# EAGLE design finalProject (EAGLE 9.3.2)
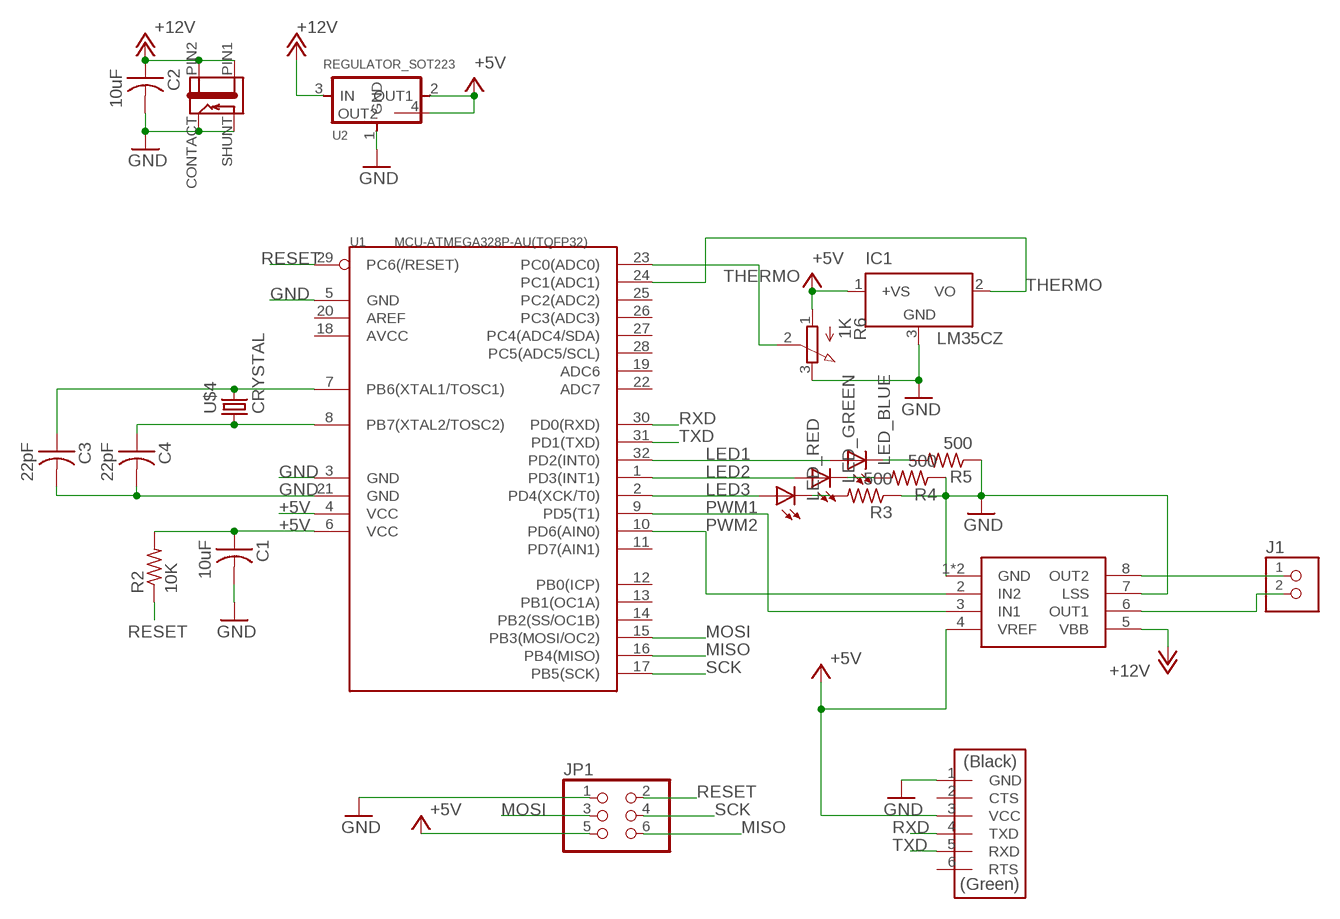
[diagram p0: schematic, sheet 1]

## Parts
C1  10uF  CAP-US1206FAB  [C1206FAB]
C2  10uF  CAP-US1206FAB  [C1206FAB]
C3  22pF  CAP-US1206FAB  [C1206FAB]
C4  22pF  CAP-US1206FAB  [C1206FAB]
IC1  LM35CZ  [TO92]
J1  TERM-1X02-FABLAB  [ED555DS-2DS]
J2  JACK-2.1MM  [PJ-002AH-SMT]
JP1  PINHD-2X3-SMD  [2X03SMD]
LED_BLUE  LEDFAB1206  [LED1206FAB]
LED_GREEN  LEDFAB1206  [LED1206FAB]
LED_RED  LEDFAB1206  [LED1206FAB]
R2  10K  RES-US1206FAB  [R1206FAB]
R3  500  RES-US1206FAB  [R1206FAB]
R4  500  RES-US1206FAB  [R1206FAB]
R5  500  RES-US1206FAB  [R1206FAB]
R6  1K  3RP/1610N  [3RP/1610N]
U1  MCU-ATMEGA328P-AU(TQFP32)  [TQFP32-0.8-7X7MM]
U2  REGULATOR_SOT223  [SOT223]
U$1  A4953-H-BRIDGE-MOTOR-DRIVER-PAD  [SOIC8_PAD]
U$2  FTDI-SMD-HEADER  [1X06SMD]
U$4  CRYSTAL  [2-SMD-5X3MM]

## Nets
+5V: C1.1 IC1.1(+VS) JP1.5 R2.2 R6.1(A) U1.4(VCC) U1.6(VCC) U2.2(OUT1) U2.4(OUT2) U$1.4(VREF) U$2.3(VCC)
+12V: C2.1 J2.PIN1 J2.PIN2 U2.3(IN) U$1.5(VBB)
GND: C1.2 C2.2 C3.2 C4.2 IC1.3(GND) J2.CONTACT J2.SHUNT JP1.1 R3.1 R4.1 R5.1 R6.3(E) U1.3(GND) U1.5(GND) U1.21(GND) U2.1(GND) U$1.1(GND) U$1.7(LSS) U$1.GND U$2.1(GND)
LED1: LED_BLUE.1(A) U1.32(PD2(INT0))
LED2: LED_GREEN.1(A) U1.1(PD3(INT1))
LED3: LED_RED.1(A) U1.2(PD4(XCK/T0))
MISO: JP1.6 U1.16(PB4(MISO))
MOSI: JP1.3 U1.15(PB3(MOSI/OC2))
N$1: R6.2(S) U1.23(PC0(ADC0))
N$2: LED_RED.2(C) R3.2
N$3: LED_BLUE.2(C) R5.2
N$4: C3.1 U1.7(PB6(XTAL1/TOSC1)) U$4.P$2
N$5: C4.1 U1.8(PB7(XTAL2/TOSC2)) U$4.P$1
N$6: LED_GREEN.2(C) R4.2
N$7: J1.1 U$1.8(OUT2)
N$8: J1.2 U$1.6(OUT1)
PWM1: U1.9(PD5(T1)) U$1.3(IN1)
PWM2: U1.10(PD6(AIN0)) U$1.2(IN2)
RESET: JP1.2 R2.1 U1.29(PC6(/RESET))
RXD: U1.30(PD0(RXD)) U$2.4(TXD)
SCK: JP1.4 U1.17(PB5(SCK))
THERMO: IC1.2(VO) U1.24(PC1(ADC1))
TXD: U1.31(PD1(TXD)) U$2.5(RXD)
Unconnected: U1.11(PD7(AIN1)) U1.12(PB0(ICP)) U1.13(PB1(OC1A)) U1.14(PB2(SS/OC1B)) U1.18(AVCC) U1.19(ADC6) U1.20(AREF) U1.22(ADC7) U1.25(PC2(ADC2)) U1.26(PC3(ADC3)) U1.27(PC4(ADC4/SDA)) U1.28(PC5(ADC5/SCL)) U$2.2(CTS) U$2.6(RTS)

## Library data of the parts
C1-C4 = fab:CAP-US
IC1 = lm35:LM35: Single-Supply Centigrade Temperature Sensor Vout = (10mV/°C x Temp °C) +5mmmV Source: http://www.national.com/ds/LM/LM35.pdf
J1 = fab:TERM-1X02: 3.5mm terminal block, 2 positions ED555-2DS as found in the fablab inventory.
J2 = fab:JACK-2.1MM: SMD DC power jack PJ-002AH-SMT As found in the fablab inventory. Made by Zaerc.
JP1 = fab:PINHD-2X3-SMD: PIN HEADER
LED_BLUE LED_GREEN LED_RED = fab:LED: LED
R2-R5 = fab:RES-US: Resistor (US Symbol)
R6 = pot:3RP/1610N: 16mm Potentiometer one level Source: http://www.alphapotentiometers.net/html/16mm_pot_2.html
U1 = MCU-ATMEGA328P-AU_TQFP32_:MCU-ATMEGA328P-AU(TQFP32): 310010049; AVAILABILITY: Unavailable; DESCRIPTION: Microcontroller Mcu, 8 Bit, Atmega, 20mhz, Tqfp-32; MF: Microchip; MP: ATMEGA328P-AU; PACKAGE: TQFP-32 Microchip; PRICE: None
U2 = fab:REGULATOR_SOT223
U$1 = fab:A4953-H-BRIDGE-MOTOR-DRIVER-PAD
U$2 = fab:FTDI-SMD-HEADER
U$4 = fab:CRYSTAL

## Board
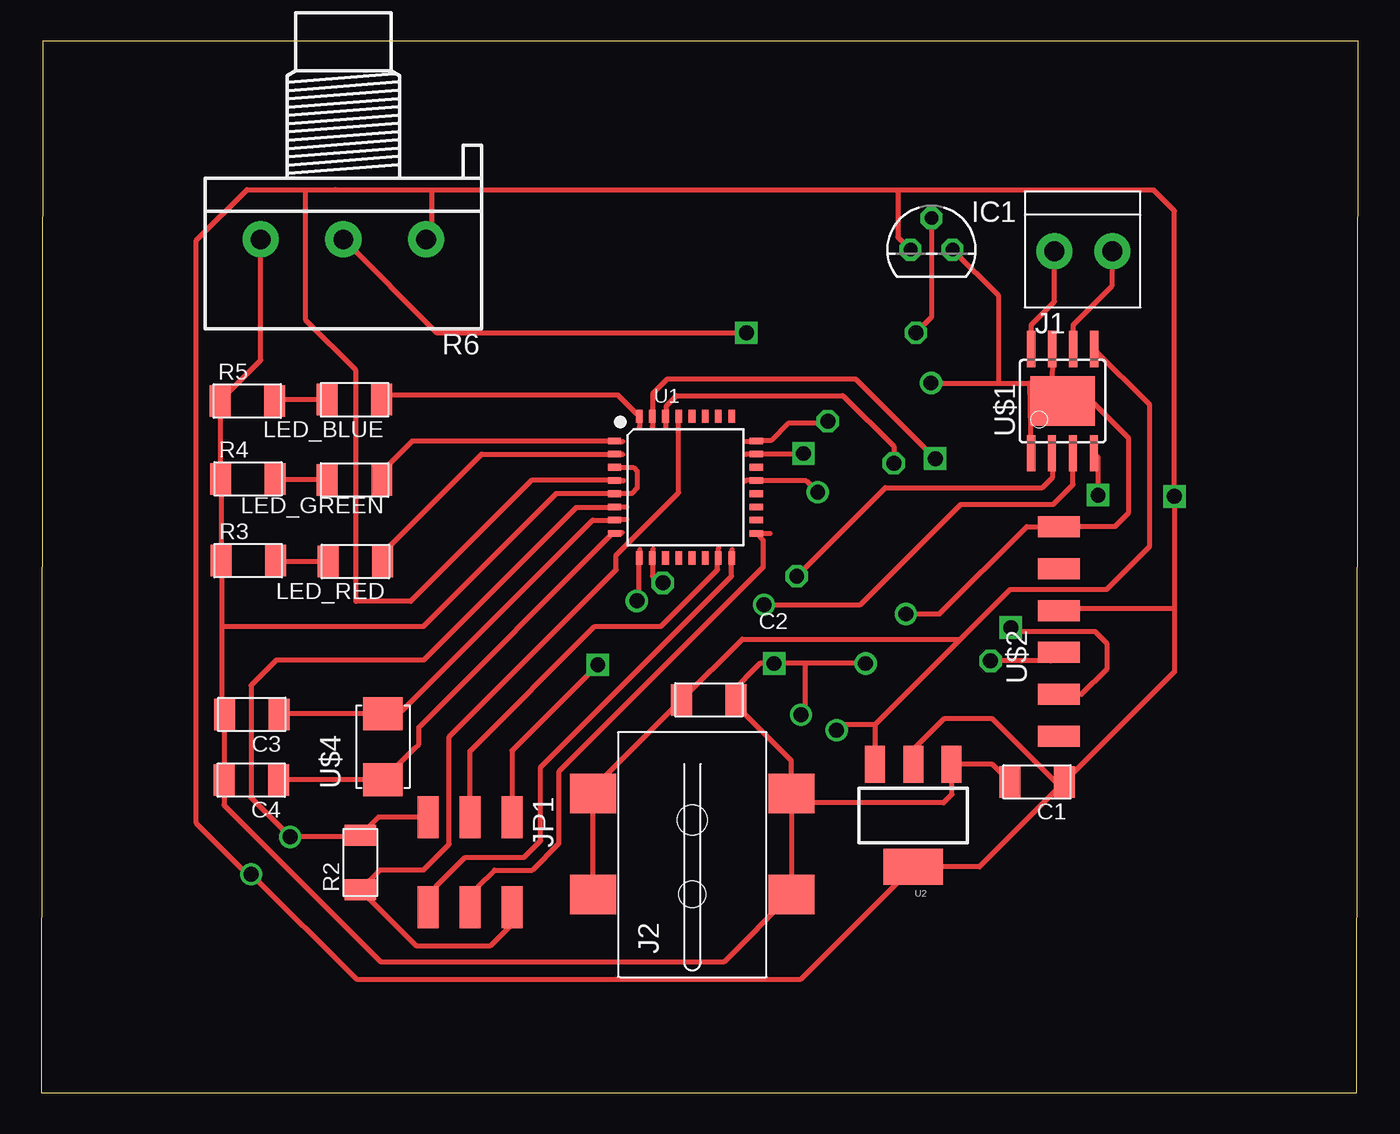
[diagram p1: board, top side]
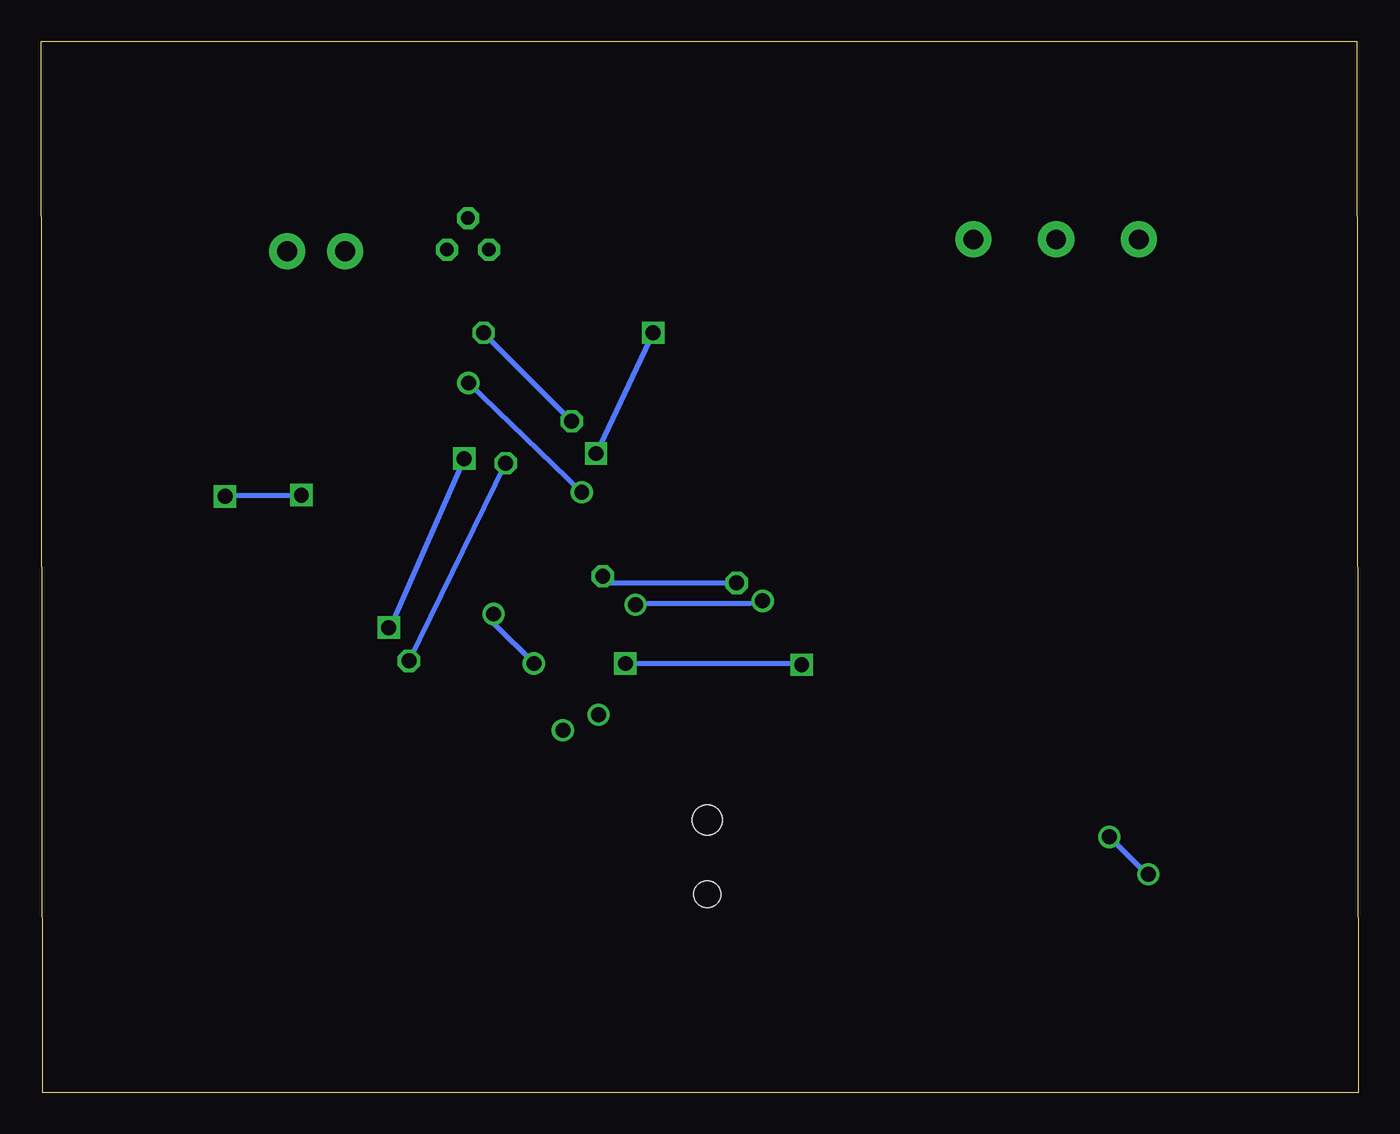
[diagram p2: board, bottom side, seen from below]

Size 79.7 x 63.6 mm. Coordinates in mm from the lower left corner, seen from the top.
Outline: 0,0 79.6,0 79.7,63.6 0.1,63.6 0,0
Copper layers (1*16): Top 0.035mm / dielectric 1.5mm / Bottom 0.035mm
Design rules "default *": minimum track width 6mil, minimum drill 0.35mm, track to track 0.4mm, track to pad 0.4mm, pad to pad 0.4mm, via to via 0.4mm, smd to smd 0.4mm, copper to edge 40mil, drill to drill 6mil, minimum pad ring 10mil, minimum via ring 8mil, stop-mask expansion 4mil, vias tented up to drill 0mil, thermal gap 10mil

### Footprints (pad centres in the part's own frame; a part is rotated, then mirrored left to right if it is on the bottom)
C1206FAB = smd 1.27 x 1.905: 1 -1.651,0; 2 1.651,0
TO92 = drill 0.813 octagon: 1 -1.27,0; 2 0,1.905; 3 1.27,0
ED555DS-2DS = drill 1.2 pad 2.184: 1 1.8,0; 2 -1.7,0
PJ-002AH-SMT = smd 2.4 x 2.8: CONTACT -2.4,-6; PIN1 3.7,6; PIN2 -2.4,6; SHUNT 3.7,-6 | hole 1.6: -2.4,0 | hole 1.8: 2.1,0
2X03SMD = smd 2.54 x 1.27: 1 -2.54,2.54; 2 2.92,2.54; 3 -2.54,0; 4 2.92,0; 5 -2.54,-2.54; 6 2.92,-2.54
LED1206FAB = smd 1.27 x 1.905: 1 -1.651,0; 2 1.651,0
R1206FAB = smd 1.27 x 1.905: 1 -1.651,0; 2 1.651,0
3RP/1610N = drill 1.2 pad 2.184: 1 -5,0; 2 0,0; 3 5,0
TQFP32-0.8-7X7MM = smd 0.8 x 0.4: 1 -4.293,2.8; 2 -4.293,2; 3 -4.293,1.2; 4 -4.293,0.4; 5 -4.293,-0.4; 6 -4.293,-1.2; 7 -4.293,-2; 8 -4.293,-2.8; 17 4.293,-2.8; 18 4.293,-2; 19 4.293,-1.2; 20 4.293,-0.4; 21 4.293,0.4; 22 4.293,1.2; 23 4.293,2; 24 4.293,2.8 | smd 0.4 x 0.8: 9 -2.8,-4.293; 10 -2,-4.293; 11 -1.2,-4.293; 12 -0.4,-4.293; 13 0.4,-4.293; 14 1.2,-4.293; 15 2,-4.293; 16 2.8,-4.293; 25 2.8,4.293; 26 2,4.293; 27 1.2,4.293; 28 0.4,4.293; 29 -0.4,4.293; 30 -1.2,4.293; 31 -2,4.293; 32 -2.8,4.293
SOT223 = smd 1.219 x 2.235: 1 -2.311,-3.099; 2 0,-3.099; 3 2.311,-3.099 | smd 3.6 x 2.2: 4 0,3.099
SOIC8_PAD = smd 0.5 x 2.2: 1 -1.905,-3.154; 2 -0.645,-3.154; 3 0.625,-3.154; 4 1.895,-3.154; 5 1.905,3.154; 6 0.635,3.154; 7 -0.635,3.154; 8 -1.905,3.154 | smd 3.886 x 2.997: GND 0,0
1X06SMD = smd 2.54 x 1.27: 1 0,6.35; 2 0,3.81; 3 0,1.27; 4 0,-1.27; 5 0,-3.81; 6 0,-6.35
2-SMD-5X3MM = smd 2 x 2.4: P$1 -2,0; P$2 2,0

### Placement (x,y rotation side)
C1  60.26,18.79 180 top
C2  40.4,23.76 0 top
C3  12.74,22.88 180 top
C4  12.71,18.9 180 top
IC1  53.87,50.99 0 top
J1  63.12,50.9 180 top
J2  39.4,14.39 90 top
JP1  25.94,14.12 270 top
LED_BLUE  18.96,41.92 180 top
LED_GREEN  18.96,37.06 180 top
LED_RED  19.01,32.13 180 top
R2  19.31,13.91 90 top
R3  12.52,32.19 0 top
R4  12.51,37.13 0 top
R5  12.47,41.84 0 top
R6  18.28,51.61 180 top
U1  38.98,36.63 0 top
U2  52.77,16.76 180 top
U$1  61.81,41.83 0 top
U$2  61.58,27.89 0 top
U$4  20.68,20.92 90 top

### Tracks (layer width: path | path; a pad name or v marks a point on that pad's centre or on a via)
+5V  (via drill 0.9)
  Top 0.305: IC1.1 51.84,51.76 51.84,54.61 23.62,54.61 | U2.2 52.6,20.02 52.6,20.57 54.64,22.61 57.57,22.61 61.38,18.79 C1.1 | JP1.5 20.4,16.66 R2.2 | C1.1 56.78,13.66 U2.4 45.97,6.86 19.07,6.86 v12.71,13.22 | 17.78,54.61 17.8,54.63 12.45,54.63 9.38,51.56 9.38,16.3 12.46,13.22 v12.71,13.22 | 17.78,54.61 16,54.61 16,46.74 19.05,43.69 19.05,29.72 22.35,29.72 29.66,37.03 U1.4 35.21,37.03 35.23,37.01 | 17.78,54.61 23.62,54.61 | 23.62,54.61 23.62,51.95 R6.1 | 51.59,54.61 67.31,54.61 68.58,53.34 v68.58,36.07 68.58,29.29 | C1.1 68.58,25.46 68.58,29.29 | U$2.3 61.71,29.29 68.58,29.29 | U$1.4 63.96,38.43 v63.96,36.14 | 19.11,15.37 R2.2 | 19.24,15.49 R2.2 | v12.7,13.21 v12.71,13.22 | R2.2 19.21,15.47 v15.06,15.47 12.7,17.83 12.7,24.64 14.22,26.16 23.14,26.16 32.36,35.38 34.64,35.38 U1.6 35.43,35.43
  Bottom 0.305: v68.58,36.07 68.5,36.14 v63.96,36.14 | v15.06,15.47 12.8,13.21 v12.7,13.21
+12V  (via drill 0.9)
  Top 0.305: J2.PIN2 J2.PIN1 33.4,18.41 C2.1 42.42,27.43 55.63,27.43 | U$1.5 67.06,41.65 67.06,33.02 64.47,30.43 58.62,30.43 55.63,27.43 | 50.46,22.27 U2.3 | 55.63,27.43 50.46,22.27 | 50.46,22.27 48.48,22.27 v48.13,21.92
GND  (via drill 0.9)
  Top 0.305: 11.06,22.85 C3.2 11.19,22.78 | 11.06,22.85 C4.2 11.06,17.39 20.52,7.92 41.34,7.92 J2.CONTACT | R6.3 13.28,44.3 R5.1 10.86,41.8 R4.1 10.87,37.12 R3.1 10.92,32.13 10.92,28.19 | IC1.3 57.91,48.23 57.91,42.93 | J2.SHUNT 45.4,20.08 41.88,23.6 C2.2 | C2.2 41.67,24.14 43.48,25.96 v44.35,25.96 44.37,25.98 46.23,25.98 | C2.2 | J2.CONTACT 44.54,12.85 | U2.1 55.48,19.86 | U2.1 55.12,19.82 55.12,18.03 54.61,17.53 45.96,17.53 J2.SHUNT | U$2.1 61.38,34.04 | 11.06,22.85 10.92,22.99 10.92,28.19 | 10.92,28.19 23.11,28.19 31.15,36.23 U1.5 35.72,36.23 36.07,36.58 36.07,37.59 35.83,37.83 U1.3 | C1.2 57.55,19.86 U2.1 | 59.94,38.71 U$1.1 59.82,42.93 | U$2.1 64.98,34.24 65.79,35.05 65.79,39.62 63.75,41.66 | 63.58,41.83 63.75,41.66 | J2.SHUNT J2.CONTACT | JP1.1 28.48,20.69 v33.68,25.88 | U$2.1 59.64,34.24 54.36,28.96 v52.32,28.96 | v46.99,36.32 46.31,37.01 43.3,37.01 U1.21 42.67,37.03 42.65,37.01 | v49.89,25.96 49.86,25.98 46.23,25.98 | v53.85,42.93 57.91,42.93 | 57.91,42.93 59.82,42.93 | 59.82,42.93 60.45,42.93 U$1.GND 61.16,42.35 | U$1.7 61.16,42.35 | 61.16,42.35 63.75,41.66 | 46.23,25.98 46.23,23.11 v45.97,22.86
  Bottom 0.305: v44.35,25.96 33.76,25.96 v33.68,25.88 | v52.32,28.96 52.32,28.4 v49.89,25.96 | v46.99,36.32 v53.85,42.93
LED1
  Top 0.305: LED_BLUE.1 20.89,42.19 34.91,42.19 U1.32 36.2,40.91 36.2,40.26
LED2
  Top 0.305: LED_GREEN.1 20.61,37.57 22.47,39.43 U1.1 34.73,39.38 35.18,39.38
LED3
  Top 0.305: LED_RED.1 20.66,32.64 26.65,38.63 U1.2 35.16,38.63 35.18,38.61
MISO
  Top 0.305: JP1.6 23.88,11.67 23.88,12.45 25.65,14.22 29.21,14.22 30.23,15.24 30.23,19.68 41.78,31.24 U1.16 41.81,32.37 41.81,32.87
MOSI
  Top 0.305: JP1.3 25.94,20.66 33.49,28.21 37.51,28.21 40.93,31.63 40.93,32.29 U1.15 40.98,32.93 41,32.94
N$1  (via drill 0.9)
  Top 0.305: R6.2 23.92,45.97 v42.67,45.97 | v46.13,38.66 46.1,38.63 U1.23 42.69,38.63 42.67,38.61
  Bottom 0.305: v42.67,45.97 v46.13,38.66
N$2
  Top 0.305: LED_RED.2 14.23,32.13 R3.2
N$3
  Top 0.305: LED_BLUE.2 14.2,41.92 R5.2
N$4
  Top 0.305: C3.1 14.43,22.92 U$4.P$2 20.87,23.11 21.85,23.11 33.37,34.63 U1.7 34.73,34.67 35.43,34.67
N$5
  Top 0.305: C4.1 14.38,18.92 U$4.P$1 22.59,20.83 22.61,20.83 22.86,21.08 22.86,22.11 34.58,33.83 U1.8 35.1,33.83 35.15,33.88 35.17,33.88
N$6
  Top 0.305: LED_GREEN.2 14.23,37.06 R4.2
N$7
  Top 0.305: U$1.8 59.91,46.45 61.32,47.86 J1.1
N$8
  Top 0.305: U$1.6 62.45,46.45 64.82,48.82 J1.2
PWM1  (via drill 0.9)
  Top 0.305: v43.74,29.52 49.58,29.52 55.65,35.59 61.24,35.59 62.44,36.78 U$1.3 | v36.04,29.74 36.14,29.84 36.14,32.3 U1.9 36.18,32.75 36.23,32.8 36.23,32.84
  Bottom 0.305: v43.74,29.52 43.66,29.59 36.83,29.59 v36.04,29.74
PWM2  (via drill 0.9)
  Top 0.305: v37.62,30.84 37.38,30.84 36.98,31.24 U1.10 37.03,32.38 37.03,32.89 | v45.72,31.24 51.08,36.6 60.58,36.6 61.21,37.24 61.21,38.63 U$1.2
  Bottom 0.305: v45.72,31.24 45.31,30.84 v37.62,30.84
RESET
  Top 0.305: JP1.2 28.48,10.2 27.18,8.89 22.68,8.89 R2.1 20.51,13.46 23.11,13.46 24.69,15.04 24.69,21.51 34.8,31.62 34.8,32.51 38.58,36.29 U1.29
RXD  (via drill 0.9)
  Top 0.305: U$2.4 61.08,26.12 v57.45,26.12 | v51.59,38.07 51.59,39.09 48.51,42.16 38.44,42.16 37.83,41.55 37.83,40.97 U1.30 37.78,40.25 37.8,40.23
  Bottom 0.305: v51.59,38.07 v57.45,26.12
SCK
  Top 0.305: JP1.4 26.42,11.67 26.42,12.45 27.43,13.46 29.72,13.46 31.32,15.06 31.32,19.41 43.69,31.78 43.69,33.41 U1.17 44.12,33.83
THERMO  (via drill 0.9)
  Top 0.305: IC1.2 53.87,46.91 v52.93,45.97 | v47.6,40.62 47.6,40.49 45.2,40.49 44.2,39.48 43.32,39.48 U1.24 43.22,39.38 42.67,39.38
  Bottom 0.305: v52.93,45.97 52.93,45.95 v47.6,40.62
TXD  (via drill 0.9)
  Top 0.305: U$2.5 62.95,24.08 64.52,25.65 64.52,27.15 63.78,27.89 58.92,27.89 v58.67,28.13 | v54.1,38.35 49.28,43.18 37.89,43.18 37.03,42.31 37.03,40.97 U1.31 36.98,40.29 37.01,40.26
  Bottom 0.305: v54.1,38.35 58.67,27.94 v58.67,28.13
